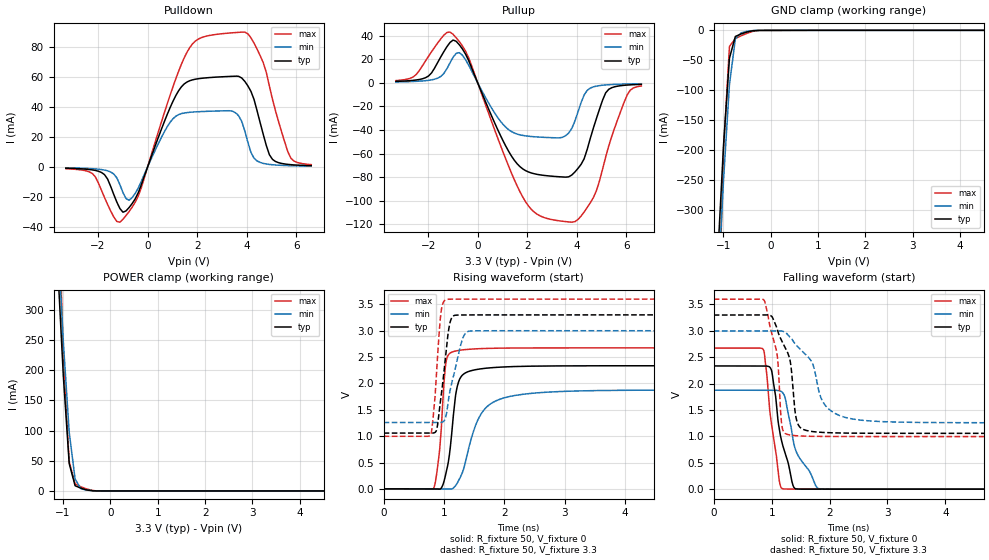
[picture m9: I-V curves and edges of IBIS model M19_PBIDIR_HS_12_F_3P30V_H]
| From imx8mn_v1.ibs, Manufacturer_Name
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[Model] M19_PBIDIR_HS_12_F_3P30V_H
Model_type I/O
Vinl  =  0.99
Vinh  =  2.31
Vmeas =  1.65
| Capacitance   typ   min   max
C_comp   1.08818991111e-12   1.03117834871e-12   1.10439570077e-12
| Variables   typ   min   max
[GND Clamp Reference]   0   0   0
[POWER Clamp Reference]   3.3   3   3.6
[Pulldown Reference]   0   0   0
[Pullup Reference]   3.3   3   3.6
[Temperature Range]   25   125   -40
[Voltage Range]   3.3   3   3.6
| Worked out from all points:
|   slope of the pulldown table from 0 to 0.495 V, typ, clamps not added: 22.1 ohm
|   slope of the pullup table from 0 to 0.495 V, typ, clamps not added: 19.9 ohm
|   GND clamp passes 1 mA (typ) near -0.39 V on its own axis
|   POWER clamp passes 1 mA (typ) near -0.44 V on its own axis
|   falling waveform, R_fixture 50, V_fixture 0: 20-80 % time 238ps typ, 359ps min, 173ps max; typ from 2.34 V to 0.002 V
|   falling waveform, R_fixture 50, V_fixture 3.3: 20-80 % time 244ps typ, 419ps min, 179ps max; typ from 3.3 V to 1.06 V
|   rising waveform, R_fixture 50, V_fixture 0: 20-80 % time 141ps typ, 341ps min, 100ps max; typ from 0.002 V to 2.34 V
|   rising waveform, R_fixture 50, V_fixture 3.3: 20-80 % time 133ps typ, 195ps min, 94ps max; typ from 1.06 V to 3.3 V
[GND Clamp]
| Voltage   I(typ)   I(min)   I(max)
-3.3V     -7.236A    -6.565A    -8.004A
-1.117V   -380.4mA   -438.7mA   -546.7mA
-993.1mV  -191mA     -249.4mA   -198.9mA
-869mV    -46.61mA   -90.79mA   -26.93mA
-744.8mV  -10.31mA   -14.37mA   -13.71mA
-620.7mV  -5.945mA   -4.193mA   -9.059mA
-372.4mV  -659.7uA   -360.2uA   -1.673mA
-248.3mV  -143.8uA   -94.2uA    -265.5uA
6.6V      0A         0A         0A
[POWER Clamp]
| Voltage   I(typ)   I(min)   I(max)
-3.3V     7.237A     6.564A     8.009A
-1.117V   380.7mA    433.6mA    553.5mA
-993.1mV  190.7mA    247mA      219.9mA
-869mV    45.33mA    97.36mA    48.38mA
-744.8mV  8.677mA    19.82mA    11.82mA
-620.7mV  4.425mA    3.499mA    6.828mA
-372.4mV  215.5uA    293.3uA    764.6uA
-248.3mV  4.273uA    22.4uA     51.08uA
6.6V      0A         0A         0A
[Pulldown]
| Voltage   I(typ)   I(min)   I(max)
-3.3V     -840.9uA   -581.7uA   -1.166mA
-2.234V   -1.962mA   -1.161mA   -4.306mA
-1.738V   -5.114mA   -2.084mA   -20.29mA
-1.117V   -27.64mA   -11.77mA   -36.7mA
-620.7mV  -24.27mA   -20.33mA   -26.65mA
910.3mV   39.51mA    29.7mA     47.83mA
1.707V    57.32mA    36.31mA    79.47mA
3.797V    59.08mA    30.26mA    89.55mA
4.293V    44.81mA    5.808mA    82.22mA
5.038V    5.003mA    1.452mA    44.86mA
5.783V    1.505mA    808.7uA    5.722mA
6.6V      854.3uA    541.3uA    1.528mA
[Pullup]
| Voltage   I(typ)   I(min)   I(max)
-3.3V     1.292mA    812.3uA    1.969mA
-2.607V   2.182mA    1.225mA    5.027mA
-1.986V   5.844mA    2.197mA    22.58mA
-993.1mV  36.41mA    21.83mA    41.25mA
-620.7mV  28.92mA    23.62mA    31.49mA
1.024V    -49.28mA   -35.28mA   -58.9mA
1.934V    -74.55mA   -44.98mA   -101.1mA
3.797V    -78.17mA   -38.58mA   -118.3mA
4.417V    -56.34mA   -6.331mA   -105.8mA
5.162V    -8.389mA   -1.702mA   -62.83mA
6.031V    -1.815mA   -906.2uA   -10.09mA
6.6V      -1.22mA    -691.9uA   -2.554mA
[Ramp]
dV/dt_r   1.4006/0.141063n  1.1252/0.340599n  1.60348/0.100285n
dV/dt_f   1.34487/0.244231n  1.04489/0.418706n  1.56141/0.179352n
R_load = 50
[Falling Waveform]
R_fixture = 50
V_fixture = 0
V_fixture_min = 0
V_fixture_max = 0
| Time   V(typ)   V(min)   V(max)
0s        2.336V     1.876V     2.675V
859.9ps   2.336V     1.876V     2.637V
1.001ns   2.239V     1.876V     1.208V
1.129ns   1.151V     1.866V     177.8mV
1.251ns   620.9mV    1.634V     3.174mV
1.367ns   76.15mV    952.3mV    2.529mV
1.435ns   4.912mV    685.7mV    2.529mV
1.775ns   1.798mV    43.02mV    2.529mV
1.935ns   1.746mV    1.728mV    2.528mV
333.3ns   1.508mV    1.043mV    2.062mV
[Falling Waveform]
R_fixture = 50
V_fixture = 3.3
V_fixture_min = 3
V_fixture_max = 3.6
| Time   V(typ)   V(min)   V(max)
0s        3.3V       3V         3.6V
872.1ps   3.301V     3V         3.577V
1.093ns   3.042V     3.001V     2.562V
1.199ns   2.757V     2.99V      1.102V
1.322ns   2.418V     2.876V     1.026V
1.454ns   1.235V     2.696V     1.011V
1.705ns   1.092V     2.384V     1.002V
1.873ns   1.076V     1.68V      999.8mV
4.702ns   1.059V     1.259V     997.7mV
333.3ns   1.059V     1.259V     997.7mV
[Rising Waveform]
R_fixture = 50
V_fixture = 0
V_fixture_min = 0
V_fixture_max = 0
| Time   V(typ)   V(min)   V(max)
0s        1.508mV    1.043mV    2.062mV
828.1ps   152.1uV    1.042mV    10.26mV
928.5ps   -4.649mV   862.5uV    746.1mV
1.022ns   240.9mV    -1.752mV   2.303V
1.086ns   613mV      -3.744mV   2.561V
1.194ns   1.787V     63.67mV    2.615V
1.289ns   2.137V     266mV      2.634V
1.644ns   2.282V     1.47V      2.662V
2.237ns   2.323V     1.783V     2.672V
333.3ns   2.336V     1.876V     2.675V
[Rising Waveform]
R_fixture = 50
V_fixture = 3.3
V_fixture_min = 3
V_fixture_max = 3.6
| Time   V(typ)   V(min)   V(max)
0s        1.059V     1.259V     997.7mV
778.8ps   1.058V     1.258V     1.027V
829.1ps   1.061V     1.258V     1.461V
877.8ps   1.12V      1.258V     2.198V
955.9ps   1.797V     1.26V      3.391V
1.071ns   2.974V     1.661V     3.597V
1.141ns   3.265V     2.064V     3.599V
1.335ns   3.299V     2.916V     3.599V
1.591ns   3.299V     2.999V     3.599V
333.3ns   3.3V       3V         3.6V
[Add Submodel]
| Submodel Name Mode
M19_PBIDIR_HS_12_F_3P30V_T_H All
